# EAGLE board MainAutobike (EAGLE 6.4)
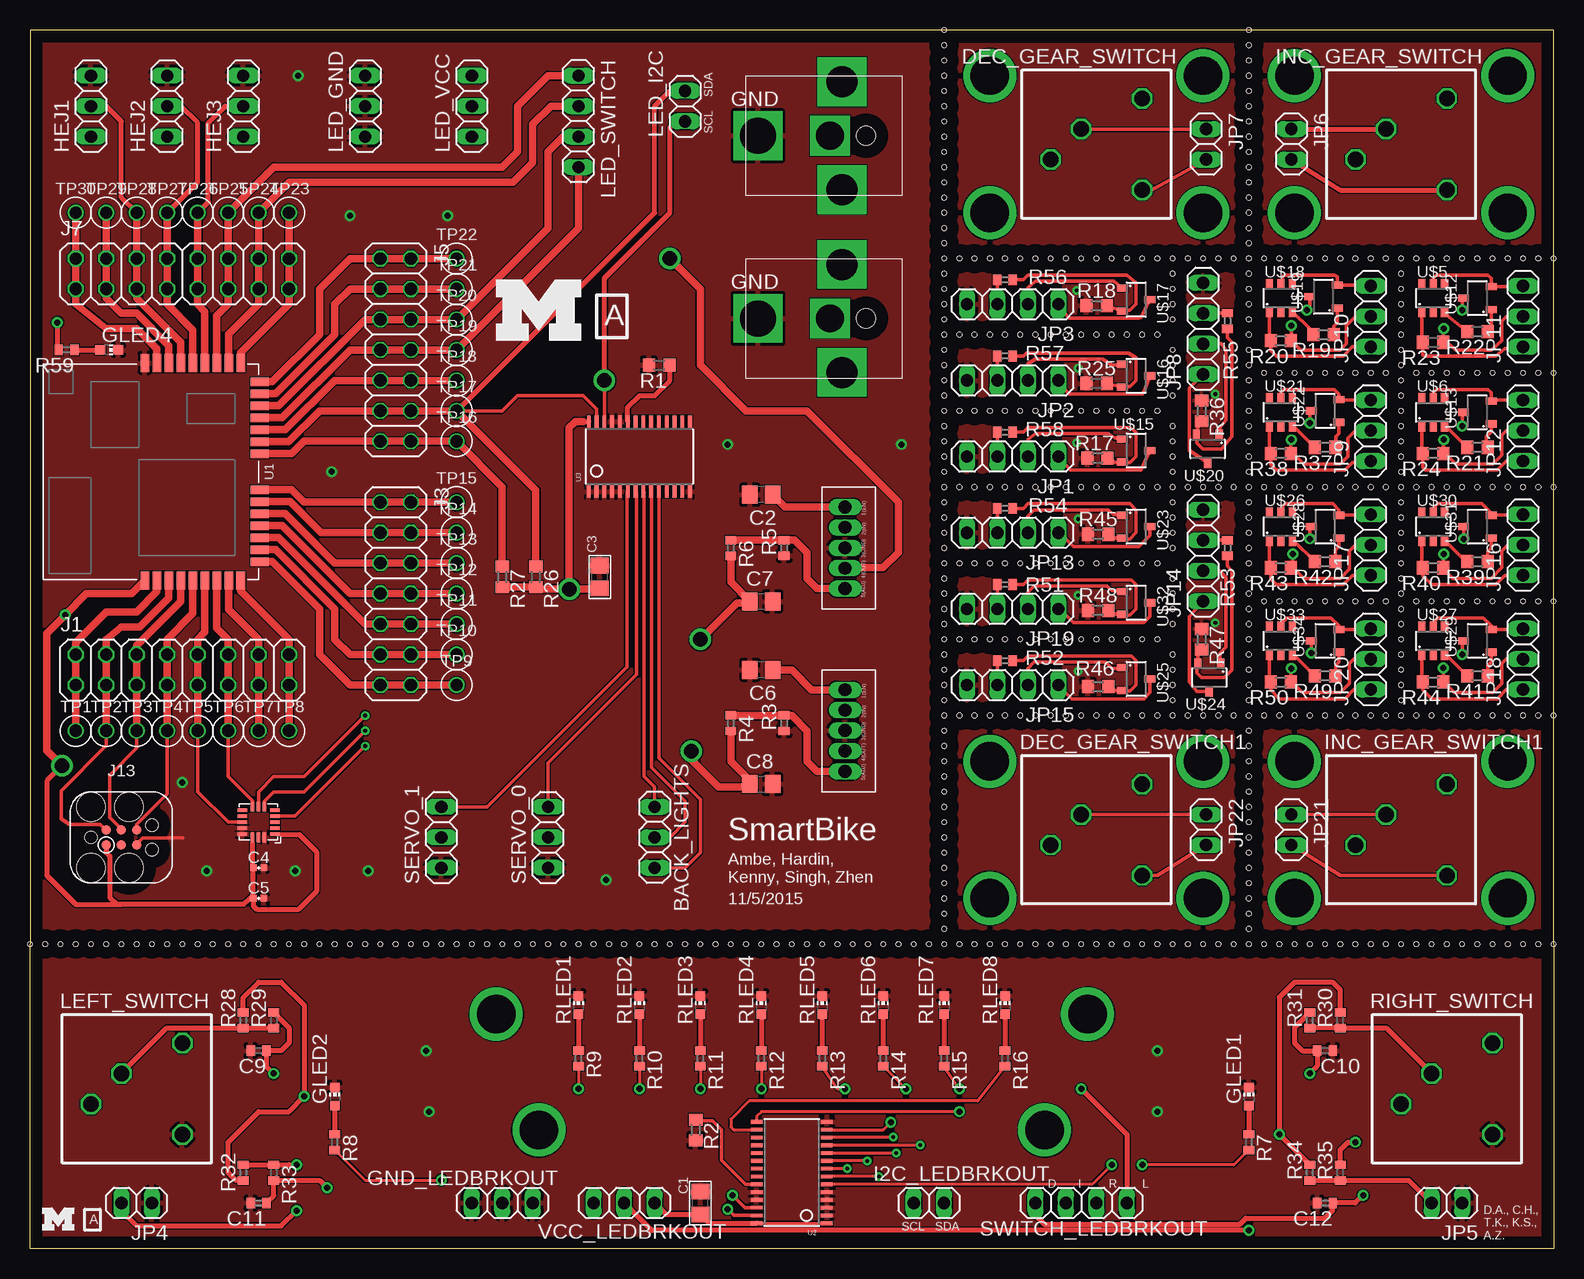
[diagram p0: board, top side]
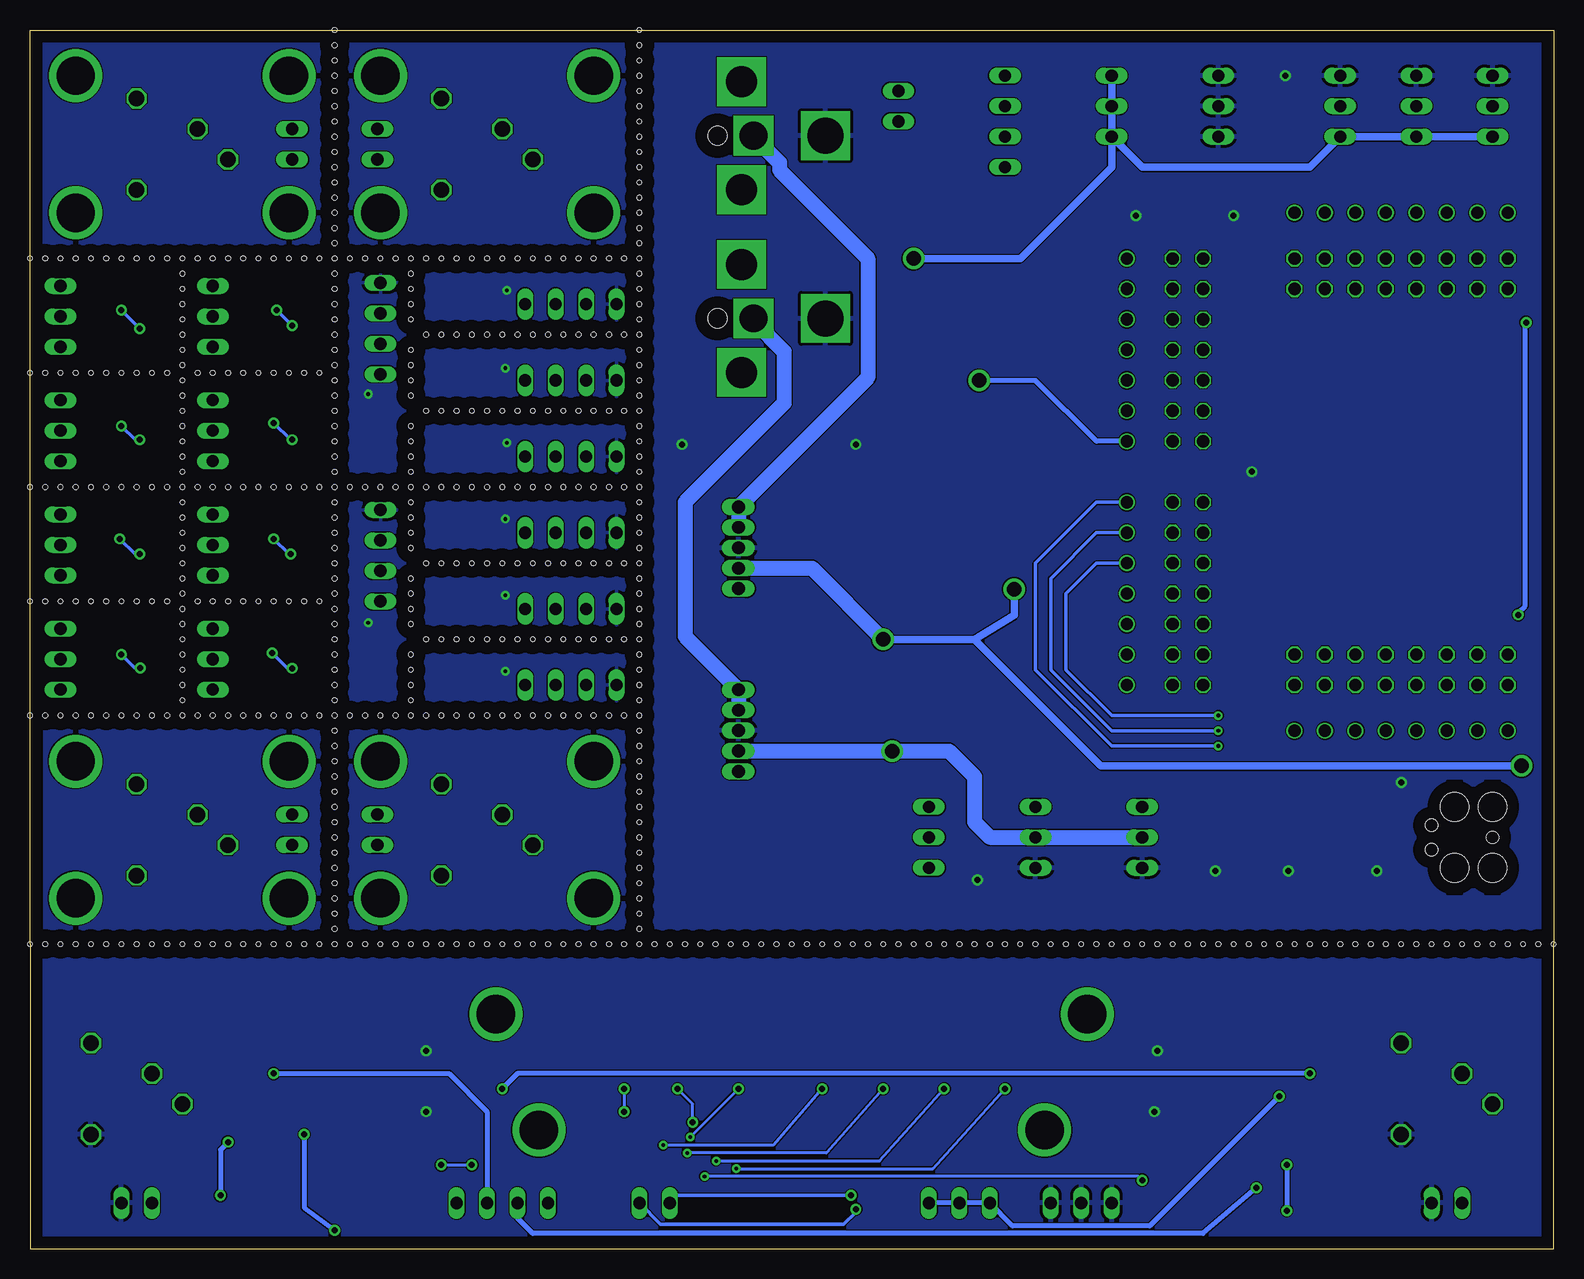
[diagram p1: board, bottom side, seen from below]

Size 127 x 101.6 mm. Coordinates in mm from the lower left corner, seen from the top.
Outline: 101.6,101.6 76.2,101.6 0,101.6 0,25.4 0,0 127,0 127,25.4 127,44.45 127,53.98 127,63.5 127,73.03 127,82.55 127,101.6 101.6,101.6
Copper layers (1*16): Top 0.035mm / dielectric 1.5mm / Bottom 0.035mm
Design rules "default *": minimum track width 4mil, minimum drill 12mil, track to track 4mil, track to pad 4mil, pad to pad 4mil, via to via 4mil, smd to smd 4mil, copper to edge 40mil, drill to drill 8mil, minimum pad ring 6mil, minimum via ring 8mil, stop-mask expansion 4mil, vias tented up to drill 0mil, thermal gap 10mil
Holes 0.38 mm at 0,25.4 1.27,25.4 2.54,25.4 3.81,25.4 5.08,25.4 6.35,25.4 7.62,25.4 8.89,25.4 10.16,25.4 11.43,25.4 12.7,25.4 13.97,25.4 15.24,25.4 16.51,25.4 17.78,25.4 19.05,25.4 20.32,25.4 21.59,25.4 22.86,25.4 24.13,25.4 25.4,25.4 26.67,25.4 27.94,25.4 29.21,25.4 30.48,25.4 31.75,25.4 33.02,25.4 34.29,25.4 35.56,25.4 36.83,25.4 38.1,25.4 39.37,25.4 40.64,25.4 41.91,25.4 43.18,25.4 44.45,25.4 45.72,25.4 46.99,25.4 48.26,25.4 49.53,25.4 50.8,25.4 52.07,25.4 53.34,25.4 54.61,25.4 55.88,25.4 57.15,25.4 58.42,25.4 59.69,25.4 60.96,25.4 62.23,25.4 63.5,25.4 64.77,25.4 66.04,25.4 67.31,25.4 68.58,25.4 69.85,25.4 71.12,25.4 72.39,25.4 73.66,25.4 74.93,25.4 76.2,25.4 77.47,25.4 78.74,25.4 80.01,25.4 81.28,25.4 82.55,25.4 83.82,25.4 85.09,25.4 86.36,25.4 87.63,25.4 88.9,25.4 90.17,25.4 91.44,25.4 92.71,25.4 93.98,25.4 95.25,25.4 96.52,25.4 97.79,25.4 99.06,25.4 100.33,25.4 101.6,25.4 102.87,25.4 104.14,25.4 105.41,25.4 106.68,25.4 107.95,25.4 109.22,25.4 110.49,25.4 111.76,25.4 113.03,25.4 114.3,25.4 115.57,25.4 116.84,25.4 118.11,25.4 119.38,25.4 120.65,25.4 121.92,25.4 123.19,25.4 124.46,25.4 125.73,25.4 127,25.4 76.2,101.6 76.2,100.33 76.2,99.06 76.2,97.79 76.2,96.52 76.2,95.25 76.2,93.98 76.2,92.71 76.2,91.44 76.2,90.17 76.2,88.9 76.2,87.63 76.2,86.36 76.2,85.09 76.2,83.82 76.2,82.55 76.2,81.28 76.2,80.01 76.2,78.74 76.2,77.47 76.2,76.2 76.2,74.93 76.2,73.66 76.2,72.39 76.2,71.12 76.2,69.85 76.2,68.58 76.2,67.31 76.2,66.04 76.2,64.77 76.2,63.5 76.2,62.23 76.2,60.96 76.2,59.69 76.2,58.42 76.2,57.15 76.2,55.88 76.2,54.61 76.2,53.34 76.2,52.07 76.2,50.8 76.2,49.53 76.2,48.26 76.2,46.99 76.2,45.72 76.2,44.45 76.2,43.18 76.2,41.91 76.2,40.64 76.2,39.37 76.2,38.1 76.2,36.83 76.2,35.56 76.2,34.29 76.2,33.02 76.2,31.75 76.2,30.48 76.2,29.21 76.2,27.94 76.2,26.67 101.6,101.6 101.6,100.33 101.6,99.06 101.6,97.79 101.6,96.52 101.6,95.25 101.6,93.98 101.6,92.71 101.6,91.44 101.6,90.17 101.6,88.9 101.6,87.63 101.6,86.36 101.6,85.09 101.6,83.82 101.6,81.28 101.6,80.01 101.6,78.74 101.6,77.47 101.6,76.2 101.6,74.93 101.6,73.66 101.6,72.39 101.6,71.12 101.6,69.85 101.6,68.58 101.6,67.31 101.6,66.04 101.6,64.77 101.6,63.5 101.6,62.23 101.6,60.96 101.6,59.69 101.6,58.42 101.6,57.15 101.6,55.88 101.6,54.61 101.6,53.34 101.6,52.07 101.6,50.8 101.6,49.53 101.6,48.26 101.6,46.99 101.6,45.72 101.6,44.45 101.6,43.18 101.6,41.91 101.6,40.64 101.6,39.37 101.6,38.1 101.6,36.83 101.6,35.56 101.6,34.29 101.6,33.02 101.6,31.75 101.6,30.48 101.6,29.21 101.6,27.94 101.6,26.67 77.47,44.45 78.74,44.45 80.01,44.45 81.28,44.45 82.55,44.45 83.82,44.45 85.09,44.45 86.36,44.45 87.63,44.45 88.9,44.45 90.17,44.45 91.44,44.45 92.71,44.45 93.98,44.45 95.25,44.45 96.52,44.45 97.79,44.45 99.06,44.45 100.33,44.45 102.87,44.45 104.14,44.45 105.41,44.45 106.68,44.45 107.95,44.45 109.22,44.45 110.49,44.45 111.76,44.45 113.03,44.45 114.3,44.45 115.57,44.45 116.84,44.45 118.11,44.45 119.38,44.45 120.65,44.45 121.92,44.45 123.19,44.45 124.46,44.45 125.73,44.45 77.47,63.5 78.74,63.5 80.01,63.5 81.28,63.5 82.55,63.5 83.82,63.5 85.09,63.5 86.36,63.5 87.63,63.5 88.9,63.5 90.17,63.5 91.44,63.5 92.71,63.5 93.98,63.5 95.25,63.5 96.52,63.5 97.79,63.5 99.06,63.5 100.33,63.5 102.87,63.5 104.14,63.5 105.41,63.5 106.68,63.5 107.95,63.5 109.22,63.5 110.49,63.5 111.76,63.5 113.03,63.5 114.3,63.5 115.57,63.5 116.84,63.5 118.11,63.5 119.38,63.5 120.65,63.5 121.92,63.5 123.19,63.5 124.46,63.5 125.73,63.5 101.6,82.55 77.47,82.55 78.74,82.55 80.01,82.55 81.28,82.55 82.55,82.55 83.82,82.55 85.09,82.55 86.36,82.55 87.63,82.55 88.9,82.55 90.17,82.55 91.44,82.55 92.71,82.55 93.98,82.55 95.25,82.55 96.52,82.55 97.79,82.55 99.06,82.55 100.33,82.55 102.87,82.55 104.14,82.55 105.41,82.55 106.68,82.55 107.95,82.55 109.22,82.55 110.49,82.55 111.76,82.55 113.03,82.55 114.3,82.55 115.57,82.55 116.84,82.55 118.11,82.55 119.38,82.55 120.65,82.55 121.92,82.55 123.19,82.55 124.46,82.55 125.73,82.55 77.47,69.85 78.74,69.85 80.01,69.85 81.28,69.85 82.55,69.85 83.82,69.85 85.09,69.85 86.36,69.85 87.63,69.85 88.9,69.85 90.17,69.85 91.44,69.85 92.71,69.85 93.98,69.85 95.25,67.31 95.25,66.04 95.25,64.77 95.25,71.12 95.25,72.39 95.25,73.66 95.25,74.93 95.25,68.58 93.98,76.2 95.25,77.47 95.25,78.74 95.25,80.01 95.25,81.28 77.47,76.2 78.74,76.2 80.01,76.2 81.28,76.2 82.55,76.2 83.82,76.2 85.09,76.2 86.36,76.2 87.63,76.2 88.9,76.2 90.17,76.2 91.44,76.2 92.71,76.2 102.87,73.03 104.14,73.03 105.41,73.03 106.68,73.03 107.95,73.03 109.22,73.03 110.49,73.03 111.76,73.03 113.03,73.03 114.3,81.28 114.3,80.01 114.3,78.74 114.3,77.47 114.3,76.2 114.3,74.93 114.3,73.66 115.57,73.03 116.84,73.03 118.11,73.03 119.38,73.03 120.65,73.03 121.92,73.03 123.19,73.03 124.46,73.03 125.73,73.03 114.3,72.39 114.3,71.12 114.3,69.85 114.3,68.58 114.3,67.31 114.3,66.04 114.3,64.77 114.3,62.23 114.3,60.96 114.3,59.69 114.3,58.42 114.3,57.15 114.3,55.88 114.3,54.61 114.3,53.34 114.3,52.07 114.3,50.8 114.3,49.53 114.3,48.26 114.3,46.99 114.3,45.72 102.87,53.98 104.14,53.98 105.41,53.98 106.68,53.98 107.95,53.98 109.22,53.98 110.49,53.98 111.76,53.98 113.03,53.98 115.57,53.98 116.84,53.98 118.11,53.98 119.38,53.98 120.65,53.98 121.92,53.98 123.19,53.98 124.46,53.98 125.73,53.98 95.25,48.26 95.25,46.99 95.25,45.72 95.25,52.07 95.25,53.34 95.25,54.61 95.25,55.88 95.25,49.53 95.25,58.42 95.25,59.69 95.25,60.96 95.25,62.23 77.47,57.15 78.74,57.15 80.01,57.15 81.28,57.15 82.55,57.15 83.82,57.15 85.09,57.15 86.36,57.15 87.63,57.15 88.9,57.15 90.17,57.15 91.44,57.15 92.71,57.15 93.98,57.15 77.47,50.8 78.74,50.8 80.01,50.8 81.28,50.8 82.55,50.8 83.82,50.8 85.09,50.8 86.36,50.8 87.63,50.8 88.9,50.8 90.17,50.8 91.44,50.8 92.71,50.8 93.98,50.8 127,82.55 127,73.03 127,63.5 127,53.98 127,44.45

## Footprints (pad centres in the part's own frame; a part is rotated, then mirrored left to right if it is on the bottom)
1X03 = drill 1.016 long: 1 -2.54,0; 2 0,0; 3 2.54,0
0805 = smd 1.3 x 1.5: 1 -0.95,0; 2 0.95,0
C0805 = smd 1.3 x 1.5: 1 -0.95,0; 2 0.95,0
0402_CAP = smd 0.536 x 0.546: 1 -0.433,0; 2 0.433,0
C0402 = smd 0.7 x 0.9: 1 -0.65,0; 2 0.65,0
LED_SWITCH = drill 1.3 octagon: P$1 -3.81,-1.27; P$2 -1.27,1.27; P$3 3.81,3.81; P$4 3.81,-3.81
CHIP-LED0603 = smd 0.8 x 0.8: A 0,-0.75; C 0,0.75
1X02 = drill 1.016 long: 1 -1.27,0; 2 1.27,0
2X08 = drill 1.016 octagon: 1 -8.89,-1.27; 2 -8.89,1.27; 3 -6.35,-1.27; 4 -6.35,1.27; 5 -3.81,-1.27; 6 -3.81,1.27; 7 -1.27,-1.27; 8 -1.27,1.27; 9 1.27,-1.27; 10 1.27,1.27; 11 3.81,-1.27; 12 3.81,1.27; 13 6.35,-1.27; 14 6.35,1.27; 15 8.89,-1.27; 16 8.89,1.27
2X07 = drill 1.016 octagon: 1 -7.62,-1.27; 2 -7.62,1.27; 3 -5.08,-1.27; 4 -5.08,1.27; 5 -2.54,-1.27; 6 -2.54,1.27; 7 0,-1.27; 8 0,1.27; 9 2.54,-1.27; 10 2.54,1.27; 11 5.08,-1.27; 12 5.08,1.27; 13 7.62,-1.27; 14 7.62,1.27
TC2030-IDC = smd 0.787 x 0.787: 1 -1.27,-0.635; 2 -1.27,0.635; 3 0,-0.635; 4 0,0.635; 5 1.27,-0.635; 6 1.27,0.635 | hole 2.375: -2.54,2.54; 0.635,2.54; 0.635,-2.54; -2.54,-2.54 | hole 1.016: -2.54,0; 2.54,1.016; 2.54,-1.016
1X04 = drill 1.016 long: 1 -3.81,0; 2 -1.27,0; 3 1.27,0; 4 3.81,0
R0603 = smd 1 x 1.1: 1 -0.85,0; 2 0.85,0
R0402 = smd 0.7 x 0.9: 1 -0.65,0; 2 0.65,0
TESTPOINT_0.040IN = drill 1.016: TESTPOINT 0,0
ATUM = smd 0.7 x 1.5: 1 -9.479,-9.079; 2 -8.479,-9.079; 3 -7.479,-9.079; 4 -6.479,-9.079; 5 -5.479,-9.079; 6 -4.479,-9.079; 7 -3.479,-9.079; 8 -2.479,-9.079; 24 -1.479,9.079; 25 -2.479,9.079; 26 -3.479,9.079; 27 -4.479,9.079; 28 -5.479,9.079; 29 -6.479,9.079; 30 -7.479,9.079; 31 -8.479,9.079; 32 -9.479,9.079 | smd 0.754 x 1.5: 9 -1.479,-9.079 | smd 1.5 x 0.7: 10 0.1,-7.5; 11 0.1,-6.5; 12 0.1,-5.5; 13 0.1,-4.5; 14 0.1,-3.5; 15 0.1,-2.5; 16 0.1,-1.5; 17 0.1,1.5; 18 0.1,2.5; 19 0.1,3.5; 20 0.1,4.5; 21 0.1,5.5; 22 0.1,6.5; 23 0.1,7.5
TSSOP28 = smd 0.305 x 0.991: 1 -4.225,-2.918; 2 -3.575,-2.918; 3 -2.925,-2.918; 4 -2.275,-2.918; 5 -1.625,-2.918; 6 -0.975,-2.918; 7 -0.325,-2.918; 8 0.325,-2.918; 9 0.975,-2.918; 10 1.625,-2.918; 11 2.275,-2.918; 12 2.925,-2.918; 13 3.575,-2.918; 14 4.225,-2.918; 15 4.225,2.918; 16 3.575,2.918; 17 2.925,2.918; 18 2.275,2.918; 19 1.625,2.918; 20 0.975,2.918; 21 0.325,2.918; 22 -0.325,2.918; 23 -0.975,2.918; 24 -1.625,2.918; 25 -2.275,2.918; 26 -2.925,2.918; 27 -3.575,2.918; 28 -4.225,2.918
ADXL362 = smd 0.8 x 0.3: P$1 -1.35,1; P$2 -1.35,0.5; P$3 -1.35,0; P$4 -1.35,-0.5; P$5 -1.35,-1; P$9 1.35,-1; P$10 1.35,-0.5; P$11 1.35,0; P$12 1.35,0.5; P$13 1.35,1 | smd 0.3 x 0.8: P$6 -0.5,-1.275; P$7 0,-1.275; P$8 0.5,-1.275; P$14 0.5,1.275; P$15 0,1.275; P$16 -0.5,1.275
MIC29710 = drill 1.067 pad 1.27 long: 1(EN) 1.664,1.905; 2(IN) 3.365,1.905; 3(GND) 5.067,1.905; 4(OUT) 6.769,1.905; 5(ADJ) 8.471,1.905
SOT23-6 = smd 0.6 x 0.9: 1 -0.95,-1.15; 2 0,-1.15; 3 0.95,-1.15; 4 0.95,1.15; 5 0,1.15; 6 -0.95,1.15
PJ063BH = drill 2.6 pad 4.064 square: FRAME0 0.5,8; FRAME1 9.5,8 | drill 3 pad 4.064 square: GND 5,1 | drill 2.3 pad 3.302 square: VDD 5,7 | hole 1.6: 5,10
SOT23-3 = smd 0.6 x 0.9: 1 -0.95,-1.15; 2 0.95,-1.15; 3 0,1.15

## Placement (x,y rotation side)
BACK_LIGHTS  [1X03]  52.07,34.29 270 top
C1  10uF  [0805]  55.88,3.81 90 top
C2  10uF  [C0805]  60.96,62.87 180 top
C3  10uF  [0805]  47.5,56.01 90 top
C4  100nF  [0402_CAP]  19.05,31.75 0 top
C5  100nF  [0402_CAP]  19.05,29.21 0 top
C6  10uF  [C0805]  60.96,48.26 180 top
C7  33uF  [C0805]  60.96,53.98 0 top
C8  33uF  [C0805]  60.96,38.73 0 top
C9  [C0402]  19.05,16.51 180 top
C10  [C0402]  107.95,16.51 0 top
C11  [C0402]  19.05,3.81 180 top
C12  [C0402]  107.95,3.81 180 top
DEC_GEAR_SWITCH  LED_SWITCH  [LED_SWITCH]  88.9,92.08 0 top
DEC_GEAR_SWITCH1  LED_SWITCH  [LED_SWITCH]  88.9,34.92 0 top
GLED1  [CHIP-LED0603]  101.6,12.7 0 top
GLED2  [CHIP-LED0603]  25.4,12.7 0 top
GLED4  [CHIP-LED0603]  6.6,74.93 270 top
GND_LEDBRKOUT  [1X03]  39.37,3.81 0 top
HEJ1  [1X03]  5.08,95.25 90 top
HEJ2  [1X03]  11.43,95.25 90 top
HEJ3  [1X03]  17.78,95.25 90 top
I2C_LEDBRKOUT  [1X02]  74.93,3.81 0 top
INC_GEAR_SWITCH  LED_SWITCH  [LED_SWITCH]  114.3,92.08 0 top
INC_GEAR_SWITCH1  LED_SWITCH  [LED_SWITCH]  114.3,34.92 0 top
J1  [2X08]  12.7,48.26 0 top
J3  [2X07]  30.48,54.61 270 top
J5  [2X07]  30.48,74.93 270 top
J7  [2X08]  12.7,81.28 0 top
J13  TC2030-CTX  [TC2030-IDC]  7.62,34.29 0 top
JP1  [1X04]  81.91,66.04 180 top
JP2  [1X04]  81.91,72.39 180 top
JP3  [1X04]  81.91,78.74 180 top
JP4  [1X02]  8.89,3.81 180 top
JP5  [1X02]  118.11,3.81 180 top
JP6  [1X02]  105.16,92.08 270 top
JP7  [1X02]  98.04,92.08 270 top
JP8  [1X04]  97.79,76.71 90 top
JP9  [1X03]  111.76,68.2 90 top
JP10  [1X03]  111.76,77.72 90 top
JP11  [1X03]  124.46,77.72 90 top
JP12  [1X03]  124.46,68.2 90 top
JP13  [1X04]  81.91,59.69 180 top
JP14  [1X04]  97.79,57.78 90 top
JP15  [1X04]  81.91,46.99 180 top
JP16  [1X03]  124.46,58.67 90 top
JP17  [1X03]  111.76,58.67 90 top
JP18  [1X03]  124.46,49.15 90 top
JP19  [1X04]  81.91,53.34 180 top
JP20  [1X03]  111.76,49.15 90 top
JP21  [1X02]  105.16,34.92 270 top
JP22  [1X02]  98.04,34.92 270 top
LED_GND  [1X03]  27.94,95.25 90 top
LED_I2C  [1X02]  54.61,95.25 90 top
LED_SWITCH  [1X04]  45.72,93.98 270 top
LED_VCC  [1X03]  36.83,95.25 90 top
LEFT_SWITCH  LED_SWITCH  [LED_SWITCH]  8.89,13.34 0 top
R1  10K  [R0603]  52.45,73.66 180 top
R2  10K  [R0603]  55.5,9.91 270 top
R3  26.1k  [R0402]  62.87,43.81 90 top
R4  100k  [R0402]  58.42,43.81 270 top
R5  60.4k  [R0402]  62.87,58.42 90 top
R6  100k  [R0402]  58.42,58.42 270 top
R7  60.4  [R0402]  101.6,8.89 270 top
R8  60.4  [R0402]  25.4,8.89 270 top
R9  261  [R0402]  45.72,15.88 270 top
R10  261  [R0402]  50.8,15.88 270 top
R11  261  [R0402]  55.88,15.88 270 top
R12  261  [R0402]  60.96,15.88 270 top
R13  261  [R0402]  66.04,15.88 270 top
R14  261  [R0402]  71.12,15.88 270 top
R15  261  [R0402]  76.2,15.88 270 top
R16  261  [R0402]  81.28,15.88 270 top
R17  10k  [R0603]  88.98,65.91 0 top
R18  10k  [R0603]  88.9,78.61 0 top
R19  1k  [R0603]  107.82,76.2 180 top
R20  390  [R0603]  104.27,75.69 180 top
R21  1k  [R0603]  120.65,66.8 180 top
R22  1k  [R0603]  120.65,76.45 180 top
R23  390  [R0603]  116.97,75.56 180 top
R24  390  [R0603]  116.97,66.29 180 top
R25  10k  [R0603]  88.9,72.14 0 top
R26  10k  [R0603]  42.16,56.01 270 top
R27  10k  [R0603]  39.37,56.01 270 top
R28  [R0402]  17.78,19.05 90 top
R29  [R0402]  20.32,19.05 90 top
R30  [R0402]  109.22,19.05 90 top
R31  [R0402]  106.68,19.05 90 top
R32  [R0402]  17.78,6.35 270 top
R33  [R0402]  20.32,6.35 270 top
R34  [R0402]  106.68,6.35 90 top
R35  [R0402]  109.22,6.35 90 top
R36  10k  [R0603]  97.66,69.85 270 top
R37  1k  [R0603]  107.95,66.8 180 top
R38  390  [R0603]  104.27,66.29 180 top
R39  1k  [R0603]  120.65,57.28 180 top
R40  390  [R0603]  116.97,56.77 180 top
R41  1k  [R0603]  120.65,47.75 180 top
R42  1k  [R0603]  107.95,57.28 180 top
R43  390  [R0603]  104.27,56.77 180 top
R44  390  [R0603]  116.97,47.24 180 top
R45  10k  [R0603]  89.03,59.56 0 top
R46  10k  [R0603]  89.03,46.86 0 top
R47  10k  [R0603]  97.66,50.8 270 top
R48  10k  [R0603]  89.03,53.21 0 top
R49  1k  [R0603]  107.95,47.75 180 top
R50  390  [R0603]  104.27,47.24 180 top
R51  33  [R0402]  81.28,55.37 0 top
R52  33  [R0402]  81.28,49.02 0 top
R53  33  [R0402]  99.82,58.42 270 top
R54  33  [R0402]  81.28,61.72 0 top
R55  33  [R0402]  99.82,77.34 270 top
R56  33  [R0402]  81.28,80.77 0 top
R57  33  [R0402]  81.28,74.42 0 top
R58  33  [R0402]  81.28,68.07 0 top
R59  60.4  [R0402]  3.05,74.93 180 top
RIGHT_SWITCH  LED_SWITCH  [LED_SWITCH]  118.11,13.34 0 top
RLED1  [CHIP-LED0603]  45.72,20.32 0 top
RLED2  [CHIP-LED0603]  50.8,20.32 0 top
RLED3  [CHIP-LED0603]  55.88,20.32 0 top
RLED4  [CHIP-LED0603]  60.96,20.32 0 top
RLED5  [CHIP-LED0603]  66.04,20.32 0 top
RLED6  [CHIP-LED0603]  71.12,20.32 0 top
RLED7  [CHIP-LED0603]  76.2,20.32 0 top
RLED8  [CHIP-LED0603]  81.28,20.32 0 top
SERVO_0  [1X03]  43.18,34.29 90 top
SERVO_1  [1X03]  34.29,34.29 90 top
SWITCH_LEDBRKOUT  [1X04]  87.63,3.81 0 top
TP1  TEST_POINT_0.040IN  [TESTPOINT_0.040IN]  3.81,43.18 0 top
TP2  TEST_POINT_0.040IN  [TESTPOINT_0.040IN]  6.35,43.18 0 top
TP3  TEST_POINT_0.040IN  [TESTPOINT_0.040IN]  8.89,43.18 0 top
TP4  TEST_POINT_0.040IN  [TESTPOINT_0.040IN]  11.43,43.18 0 top
TP5  TEST_POINT_0.040IN  [TESTPOINT_0.040IN]  13.97,43.18 0 top
TP6  TEST_POINT_0.040IN  [TESTPOINT_0.040IN]  16.51,43.18 0 top
TP7  TEST_POINT_0.040IN  [TESTPOINT_0.040IN]  19.05,43.18 0 top
TP8  TEST_POINT_0.040IN  [TESTPOINT_0.040IN]  21.59,43.18 0 top
TP9  TEST_POINT_0.040IN  [TESTPOINT_0.040IN]  35.56,46.99 0 top
TP10  TEST_POINT_0.040IN  [TESTPOINT_0.040IN]  35.56,49.53 0 top
TP11  TEST_POINT_0.040IN  [TESTPOINT_0.040IN]  35.56,52.07 0 top
TP12  TEST_POINT_0.040IN  [TESTPOINT_0.040IN]  35.56,54.61 0 top
TP13  TEST_POINT_0.040IN  [TESTPOINT_0.040IN]  35.56,57.15 0 top
TP14  TEST_POINT_0.040IN  [TESTPOINT_0.040IN]  35.56,59.69 0 top
TP15  TEST_POINT_0.040IN  [TESTPOINT_0.040IN]  35.56,62.23 0 top
TP16  TEST_POINT_0.040IN  [TESTPOINT_0.040IN]  35.56,67.31 0 top
TP17  TEST_POINT_0.040IN  [TESTPOINT_0.040IN]  35.56,69.85 0 top
TP18  TEST_POINT_0.040IN  [TESTPOINT_0.040IN]  35.56,72.39 0 top
TP19  TEST_POINT_0.040IN  [TESTPOINT_0.040IN]  35.56,74.93 0 top
TP20  TEST_POINT_0.040IN  [TESTPOINT_0.040IN]  35.56,77.47 0 top
TP21  TEST_POINT_0.040IN  [TESTPOINT_0.040IN]  35.56,80.01 0 top
TP22  TEST_POINT_0.040IN  [TESTPOINT_0.040IN]  35.56,82.55 0 top
TP23  TEST_POINT_0.040IN  [TESTPOINT_0.040IN]  21.59,86.36 0 top
TP24  TEST_POINT_0.040IN  [TESTPOINT_0.040IN]  19.05,86.36 0 top
TP25  TEST_POINT_0.040IN  [TESTPOINT_0.040IN]  16.51,86.36 0 top
TP26  TEST_POINT_0.040IN  [TESTPOINT_0.040IN]  13.97,86.36 0 top
TP27  TEST_POINT_0.040IN  [TESTPOINT_0.040IN]  11.43,86.36 0 top
TP28  TEST_POINT_0.040IN  [TESTPOINT_0.040IN]  8.89,86.36 0 top
TP29  TEST_POINT_0.040IN  [TESTPOINT_0.040IN]  6.35,86.36 0 top
TP30  TEST_POINT_0.040IN  [TESTPOINT_0.040IN]  3.81,86.36 0 top
U1  ATUM  [ATUM]  19.05,64.77 0 top
U2  PCA9685  [TSSOP28]  63.5,6.35 90 top
U3  PCA9685  [TSSOP28]  50.8,66.04 0 top
U4  ADXL362  [ADXL362]  19.05,35.56 180 top
U$1  [UMICH_SOLID_200MIL]  38.86,75.69 0 top
U$2  MIC29710  [MIC29710]  66.04,63.5 270 top
U$3  [UMICH_SOLID_75MIL]  1.02,1.52 0 top
U$4  MIC29710  [MIC29710]  66.04,48.26 270 top
U$5  HALLEFFECT  [SOT23-6]  116.97,79.25 0 top
U$6  HALLEFFECT  [SOT23-6]  116.97,69.72 0 top
U$11  PJ063PH  [PJ063BH]  59.69,97.79 270 top
U$12  25AA02E48-SOT-23-6  [SOT23-3]  120.65,79.25 90 top
U$13  25AA02E48-SOT-23-6  [SOT23-3]  120.65,69.72 90 top
U$14  PJ063PH  [PJ063BH]  59.69,82.55 270 top
U$15  25AA02E48-SOT-23-6  [SOT23-3]  92.2,66.55 270 top
U$16  25AA02E48-SOT-23-6  [SOT23-3]  92.2,72.77 270 top
U$17  25AA02E48-SOT-23-6  [SOT23-3]  92.2,79.12 270 top
U$18  HALLEFFECT  [SOT23-6]  104.27,79.25 0 top
U$19  25AA02E48-SOT-23-6  [SOT23-3]  107.82,79.38 90 top
U$20  25AA02E48-SOT-23-6  [SOT23-3]  98.17,66.67 180 top
U$21  HALLEFFECT  [SOT23-6]  104.27,69.72 0 top
U$22  25AA02E48-SOT-23-6  [SOT23-3]  107.95,69.85 90 top
U$23  25AA02E48-SOT-23-6  [SOT23-3]  92.2,60.2 270 top
U$24  25AA02E48-SOT-23-6  [SOT23-3]  98.3,47.62 180 top
U$25  25AA02E48-SOT-23-6  [SOT23-3]  92.2,47.5 270 top
U$26  HALLEFFECT  [SOT23-6]  104.27,60.2 0 top
U$27  HALLEFFECT  [SOT23-6]  116.97,50.67 0 top
U$28  25AA02E48-SOT-23-6  [SOT23-3]  107.95,60.2 90 top
U$29  25AA02E48-SOT-23-6  [SOT23-3]  120.65,50.67 90 top
U$30  HALLEFFECT  [SOT23-6]  116.97,60.2 0 top
U$31  25AA02E48-SOT-23-6  [SOT23-3]  120.65,60.2 90 top
U$32  25AA02E48-SOT-23-6  [SOT23-3]  92.2,53.85 270 top
U$33  HALLEFFECT  [SOT23-6]  104.27,50.67 0 top
U$34  25AA02E48-SOT-23-6  [SOT23-3]  107.95,50.67 90 top
VCC_LEDBRKOUT  [1X03]  49.53,3.81 0 top

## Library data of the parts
BACK_LIGHTS GND_LEDBRKOUT HEJ1-HEJ3 I2C_LEDBRKOUT JP1-JP22 LED_GND LED_I2C LED_SWITCH LED_VCC SERVO_0 SERVO_1 SWITCH_LEDBRKOUT VCC_LEDBRKOUT = pinhead
C1 C3 U2 U3 = microbuilder
C2 C6-C12 R1-R59 = rcl
C4 C5 = passives
DEC_GEAR_SWITCH DEC_GEAR_SWITCH1 INC_GEAR_SWITCH INC_GEAR_SWITCH1 LEFT_SWITCH RIGHT_SWITCH = led_switch
GLED1 GLED2 GLED4 RLED1-RLED8 = led
J1 J7 = pinhead; DIGIKEY: 609-3364-ND; MOUSER: 649-68602-116HLF; NEWARK: 20M2833
J3 J5 = pinhead; DIGIKEY: 609-3491-ND; MOUSER: 649-67996-114HLF; NEWARK: 30M1973
J13 = connector
TP1-TP30 = headers; DIGIKEY: 5001K-ND
U1 = atum
U4 = SparkFun-Sensors
U$1 U$3 = logos
U$2 U$4 = MIC29710_new2
U$5 U$6 U$12 U$13 U$15-U$34 = 25AA02E48
U$11 U$14 = PJ063PH

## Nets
19: LEFT_SWITCH.P$2 R28.1 R29.1
20: R30.1 R31.1 RIGHT_SWITCH.P$2
21: JP4.2 R32.1 R33.1
22: JP5.2 R34.1 R35.1
!RESET: J7.3 J7.4 TP29.TESTPOINT U1.30
AIN3: J7.13 J7.14 LED_SWITCH.2 TP24.TESTPOINT U1.25
AIN4: J7.11 J7.12 LED_SWITCH.1 TP25.TESTPOINT U1.26
AIN5: HEJ3.2 J7.9 J7.10 TP26.TESTPOINT U1.27
AIN6: HEJ2.2 J7.7 J7.8 TP27.TESTPOINT U1.28
AIN7: HEJ1.2 J7.5 J7.6 TP28.TESTPOINT U1.29
BATTERY: J7.1 J7.2 TP30.TESTPOINT U1.31
BOOTLOADER_CTRL: J7.15 J7.16 TP23.TESTPOINT U1.24
BOOTLOADER_RX: J5.3 J5.4 TP21.TESTPOINT U1.22
BOOTLOADER_TX: J5.1 J5.2 TP22.TESTPOINT U1.23
DEC_GEAR_SWITCH_OUT: C12.1 R35.2 SWITCH_LEDBRKOUT.1
DGND_USB: J3.13 J3.14 TP9.TESTPOINT U1.10
DVDD_USB: J3.7 J3.8 TP12.TESTPOINT U1.13
GND: C2.2 C3.2 C4.2 C5.2 C6.2 C7.2 C8.2 GLED4.C HEJ1.3 HEJ2.3 HEJ3.3 J13.5 LED_GND.1 LED_GND.2 LED_GND.3 R1.2 R3.1 R5.1 SERVO_0.1 SERVO_1.1 U1.32 U3.1 U3.2 U3.3 U3.4 U3.5 U3.14 U3.24 U3.25 U4.P$12 U4.P$13 U4.P$16 U$2.3(GND) U$4.3(GND) U$11.GND U$14.GND
GND_LEDBRKOUT: C1.2 C9.2 C10.2 C11.2 C12.2 GLED1.C GLED2.C GND_LEDBRKOUT.1 GND_LEDBRKOUT.2 GND_LEDBRKOUT.3 JP4.1 JP5.1 LEFT_SWITCH.P$4 R2.2 RIGHT_SWITCH.P$4 RLED1.C RLED2.C RLED3.C RLED4.C RLED5.C RLED6.C RLED7.C RLED8.C U2.2 U2.3 U2.4 U2.5 U2.14 U2.24 U2.25
GND_LGT1: JP1.4 R17.1
GND_LGT2: JP2.4 R25.1
GND_LGT3: JP3.4 R18.1
GND_LGT4: JP8.4 R36.1
GND_LGT5: JP13.4 R45.1
GND_LGT6: JP14.4 R47.1
GND_LGT7: JP15.4 R46.1
GND_LGT8: JP19.4 R48.1
HE1GND: JP10.3 U$18.5 U$19.2
HE1OUT: JP10.2 R20.1 U$19.3
HE1VIN: JP10.1 R20.2 U$18.1
HE2GND: JP11.3 U$5.5 U$12.2
HE2OUT: JP11.2 R23.1 U$12.3
HE2VIN: JP11.1 R23.2 U$5.1
HE3GND: JP12.3 U$6.5 U$13.2
HE3OUT: JP12.2 R24.1 U$13.3
HE3VIN: JP12.1 R24.2 U$6.1
HE4GND: JP9.3 U$21.5 U$22.2
HE4OUT: JP9.2 R38.1 U$22.3
HE4VIN: JP9.1 R38.2 U$21.1
HE5GND: JP16.3 U$30.5 U$31.2
HE5OUT: JP16.2 R40.1 U$31.3
HE5VIN: JP16.1 R40.2 U$30.1
HE6GND: JP17.3 U$26.5 U$28.2
HE6OUT: JP17.2 R43.1 U$28.3
HE6VIN: JP17.1 R43.2 U$26.1
HE7GND: JP18.3 U$27.5 U$29.2
HE7OUT: JP18.2 R44.1 U$29.3
HE7VIN: JP18.1 R44.2 U$27.1
HE8GND: JP20.3 U$33.5 U$34.2
HE8OUT: JP20.2 R50.1 U$34.3
HE8VIN: JP20.1 R50.2 U$33.1
I2C_SCL: J5.13 J5.14 LED_I2C.1 R27.1 TP16.TESTPOINT U1.17 U3.26
I2C_SCL_LEDBRKOUT: I2C_LEDBRKOUT.1 U2.26
I2C_SDA: J5.11 J5.12 LED_I2C.2 R26.1 TP17.TESTPOINT U1.18 U3.27
I2C_SDA_LEDBRKOUT: I2C_LEDBRKOUT.2 U2.27
INC_GEAR_SWITCH_OUT: C11.1 R33.2 SWITCH_LEDBRKOUT.2
LEFT_SWITCH_OUT: C9.1 R29.2 SWITCH_LEDBRKOUT.4
N$1: R16.1 RLED8.A
N$2: R5.2 R6.1 U$2.5(ADJ)
N$3: R3.2 R4.1 U$4.5(ADJ)
N$4: R15.1 RLED7.A
N$5: R14.1 RLED6.A
N$6: R13.1 RLED5.A
N$7: R12.1 RLED4.A
N$8: R11.1 RLED3.A
N$9: R10.1 RLED2.A
N$10: R9.1 RLED1.A
N$11: GLED2.A R8.1
N$12: GLED1.A R7.1
N$13: R37.1 U$22.1
N$14: R37.2 U$21.3
N$15: R19.1 U$19.1
N$16: R19.2 U$18.3
N$17: R39.1 U$31.1
N$18: R21.1 U$13.1
N$19: R39.2 U$30.3
N$20: R41.1 U$29.1
N$21: R21.2 U$6.3
N$22: R41.2 U$27.3
N$23: R42.1 U$28.1
N$24: R22.1 U$12.1
N$25: R22.2 U$5.3
N$26: R42.2 U$26.3
N$27: R49.1 U$34.1
N$28: R49.2 U$33.3
N$29: JP19.3 R51.1
N$30: JP15.3 R52.1
N$31: JP14.3 R53.1
N$32: JP13.3 R54.1
N$33: JP8.3 R55.1
N$34: JP3.3 R56.1
N$35: INC_GEAR_SWITCH.P$4 JP6.2
N$36: INC_GEAR_SWITCH.P$2 JP6.1
N$37: DEC_GEAR_SWITCH.P$4 JP7.2
N$38: DEC_GEAR_SWITCH.P$2 JP7.1
N$39: JP2.3 R57.1
N$42: JP1.3 R58.1
N$43: INC_GEAR_SWITCH1.P$4 JP21.2
N$44: INC_GEAR_SWITCH1.P$2 JP21.1
N$45: DEC_GEAR_SWITCH1.P$4 JP22.2
N$49: DEC_GEAR_SWITCH1.P$2 JP22.1
N$79: GLED4.A R59.1
OE: R1.1 U3.23
OE_LEDBRKOUT: R2.1 U2.23
OUT_LGT1: R17.2 R58.2 U$15.2
OUT_LGT2: R25.2 R57.2 U$16.2
OUT_LGT3: R18.2 R56.2 U$17.2
OUT_LGT4: R36.2 R55.2 U$20.2
OUT_LGT5: R45.2 R54.2 U$23.2
OUT_LGT6: R47.2 R53.2 U$24.2
OUT_LGT7: R46.2 R52.2 U$25.2
OUT_LGT8: R48.2 R51.2 U$32.2
P08: J5.9 J5.10 TP18.TESTPOINT U1.19
P09: J5.7 J5.8 LED_SWITCH.4 TP19.TESTPOINT U1.20
P10: J5.5 J5.6 LED_SWITCH.3 TP20.TESTPOINT U1.21
P17: J1.1 J1.2 TP1.TESTPOINT U1.2
P21: J1.9 J1.10 TP5.TESTPOINT U1.6 U4.P$11
P22: J1.11 J1.12 TP6.TESTPOINT U1.7 U4.P$8
P23: J1.13 J1.14 TP7.TESTPOINT U1.8
P24: J1.15 J1.16 TP8.TESTPOINT U1.9
PWM0: SERVO_1.3 U3.6
PWM0_0: R7.2 U2.6
PWM1: SERVO_0.3 U3.7
PWM1_0: R8.2 U2.7
PWM2: BACK_LIGHTS.1 U3.8
PWM2_0: R9.2 U2.8
PWM3: BACK_LIGHTS.2 U3.9
PWM3_0: R10.2 U2.9
PWM4: BACK_LIGHTS.3 U3.10
PWM4_0: R11.2 U2.10
PWM5: U3.11
PWM5_0: R12.2 U2.11
PWM6: U3.12
PWM6_0: R13.2 U2.12
PWM7: U3.13
PWM7_0: R14.2 U2.13
PWM8: U3.15
PWM8_0: R15.2 U2.15
PWM9: U3.16
PWM9_0: R16.2 U2.16
PWM10: U3.17
PWM10_0: U2.17
PWM11: U3.18
PWM11_0: U2.18
PWM12: U3.19
PWM12_0: U2.19
PWM13: U3.20
PWM13_0: U2.20
PWM14: U3.21
PWM14_0: U2.21
PWM15: U3.22
PWM15_0: U2.22
RIGHT_SWITCH_OUT: C10.1 R31.2 SWITCH_LEDBRKOUT.3
SIG_LGT1: JP1.2 U$15.1
SIG_LGT2: JP2.2 U$16.1
SIG_LGT3: JP3.2 U$17.1
SIG_LGT4: JP8.2 U$20.1
SIG_LGT5: JP13.2 U$23.1
SIG_LGT6: JP14.2 U$24.1
SIG_LGT7: JP15.2 U$25.1
SIG_LGT8: JP19.2 U$32.1
SPI_MISO: J3.5 J3.6 TP13.TESTPOINT U1.14 U4.P$7
SPI_MOSI: J3.3 J3.4 TP14.TESTPOINT U1.15 U4.P$6
SPI_SCK: J3.1 J3.2 TP15.TESTPOINT U1.16 U4.P$4
TCK: J1.5 J1.6 J13.4 TP3.TESTPOINT U1.4
TDO: J1.7 J1.8 J13.6 TP4.TESTPOINT U1.5
TMS: J1.3 J1.4 J13.2 TP2.TESTPOINT U1.3
USB_N: J3.9 J3.10 TP11.TESTPOINT U1.12
USB_P: J3.11 J3.12 TP10.TESTPOINT U1.11
VCC(3.3V): C3.1 C4.1 C5.1 C7.1 HEJ1.1 HEJ2.1 HEJ3.1 J13.1 LED_VCC.1 LED_VCC.2 LED_VCC.3 R6.2 R26.2 R27.2 R59.2 U1.1 U3.28 U4.P$1 U4.P$14 U$2.4(OUT)
VCC(6V): C8.1 R4.2 SERVO_0.2 SERVO_1.2 U$4.4(OUT)
VCC_LEDBRKOUT: C1.1 R28.2 R30.2 R32.2 R34.2 U2.1 U2.28 VCC_LEDBRKOUT.1 VCC_LEDBRKOUT.2 VCC_LEDBRKOUT.3
VCC_LGT1: JP1.1 U$15.3
VCC_LGT2: JP2.1 U$16.3
VCC_LGT3: JP3.1 U$17.3
VCC_LGT4: JP8.1 U$20.3
VCC_LGT5: JP13.1 U$23.3
VCC_LGT6: JP14.1 U$24.3
VCC_LGT7: JP15.1 U$25.3
VCC_LGT8: JP19.1 U$32.3
VDD1: C2.1 U$2.1(EN) U$2.2(IN) U$11.VDD
VDD2: C6.1 U$4.1(EN) U$4.2(IN) U$14.VDD

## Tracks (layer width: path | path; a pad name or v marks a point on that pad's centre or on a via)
19
  Top 0.406: R29.1 R28.1 11.41,18.4 LEFT_SWITCH.P$2
20
  Top 0.406: R31.1 R30.1 113.05,18.4 RIGHT_SWITCH.P$2
21  (via drill 0.5)
  Top 0.406: JP4.2 7.62,3.17 8.89,1.91 20.95,1.91 v22.23,3.17 | R32.1 R33.1 21.58,7 v22.23,6.98
  Bottom 0.406: v22.23,6.98 v22.23,3.17
22
  Top 0.406: JP5.2 114.95,5.7 R35.1 109.2,5.72 106.68,5.72 R34.1
!RESET
  Top 0.61: TP29.TESTPOINT J7.4 J7.3 6.35,79.25 7.62,77.98 8.89,77.98 11.57,75.3 U1.30
AIN3
  Top 0.61: LED_SWITCH.2 43.43,95.25 41.91,93.73 41.91,90.55 40.26,88.9 21.59,88.9 TP24.TESTPOINT J7.14 J7.13 19.05,78.74 16.57,76.26 U1.25
AIN4
  Top 0.61: LED_SWITCH.1 43.18,97.79 40.64,95.25 40.64,91.44 39.37,90.17 20.32,90.17 TP25.TESTPOINT J7.12 J7.11 16.51,78.74 15.57,77.8 U1.26
AIN5
  Top 0.406: TP26.TESTPOINT 14.86,87.25 14.86,93.85 16.26,95.25 HEJ3.2
  Top 0.61: U1.27 14.57,78.14 13.97,78.74 J7.9 J7.10 TP26.TESTPOINT
AIN6
  Top 0.406: HEJ2.2 12.57,95.25 13.97,93.85 13.97,88.9 TP27.TESTPOINT
  Top 0.61: U1.28 13.57,76.6 11.43,78.74 J7.7 J7.8 TP27.TESTPOINT
AIN7
  Top 0.406: TP28.TESTPOINT 7.62,87.63 7.62,93.98 6.35,95.25 HEJ1.2
  Top 0.61: U1.29 12.57,75.57 8.89,79.25 J7.5 J7.6 TP28.TESTPOINT
BATTERY
  Top 0.61: U1.31 10.57,75.03 8.89,76.71 6.35,76.71 3.81,78.74 J7.1 J7.2 TP30.TESTPOINT
BOOTLOADER_CTRL
  Top 0.61: U1.24 17.57,74.72 21.59,78.74 J7.15 J7.16 TP23.TESTPOINT
BOOTLOADER_RX
  Top 0.61: U1.22 20.47,71.27 25.4,76.2 25.4,78.74 26.67,80.01 J5.3 J5.4 TP21.TESTPOINT
BOOTLOADER_TX
  Top 0.61: U1.23 20.2,72.27 24.13,76.2 24.13,80.01 26.67,82.55 J5.1 J5.2 TP22.TESTPOINT
DEC_GEAR_SWITCH_OUT  (via drill 0.5)
  Top 0.406: R35.2 109.22,8.26 109.85,8.89 v110.49,8.89 | v111.12,4.45 110.49,3.81 C12.1 108.6,3.19 107.95,2.54 101.35,2.54 100.84,2.03 84.58,2.03 83.82,2.79 SWITCH_LEDBRKOUT.1
  Bottom 0.406: v110.49,8.89 111.12,8.26 v111.12,4.45
DGND_USB
  Top 0.61: U1.10 20.2,57.27 24.13,53.34 24.13,49.53 26.67,46.99 J3.13 J3.14 TP9.TESTPOINT
DVDD_USB
  Top 0.61: U1.13 21.01,60.27 26.67,54.61 J3.7 J3.8 TP12.TESTPOINT
GND  (via drill 0.5)
  Top 0.305: J13.5 8.89,33.76 9.4,34.27 12.73,34.27
  other vias: 12.7,38.86 14.73,31.5 28.19,31.5 48.01,30.73 58.17,67.06 72.64,67.06 26.67,86.11 34.8,86.11 22.35,97.79 25.15,64.77 22.1,31.5
  pour Bottom: 0,101.6 74.93,101.6 74.93,26.67 0,26.67
  pour Top: 0,101.6 74.93,101.6 74.93,26.67 0,26.67
GND_LEDBRKOUT  (via drill 0.5)
  other vias: 33.02,16.51 33.27,11.43 93.98,16.51 93.98,11.43
  pour Bottom: 0,24.13 127,24.13 127,0 0,0
  pour Top: 0,24.13 127,24.13 127,0 0,0
GND_LGT1  (via drill 0.3)
  other vias: 87.25,67.18
  pour Top: 76.71,69.34 94.49,69.34 94.49,64.14 76.71,64.14
  pour Bottom: 76.71,69.34 94.49,69.34 94.49,64.14 76.71,64.14
GND_LGT2  (via drill 0.3)
  other vias: 87.38,73.41
  pour Bottom: 76.71,75.56 94.49,75.56 94.49,70.36 76.71,70.36
  pour Top: 76.71,75.56 94.49,75.56 94.49,70.36 76.71,70.36
GND_LGT3  (via drill 0.3)
  other vias: 87.25,79.88
  pour Bottom: 76.71,81.91 94.49,81.91 94.49,76.96 76.71,76.96
  pour Top: 76.71,81.91 94.49,81.91 94.49,76.96 76.71,76.96
GND_LGT4  (via drill 0.3)
  other vias: 98.81,71.25
  pour Bottom: 95.63,82.17 100.97,82.17 100.97,64.26 95.63,64.26
  pour Top: 95.63,82.17 100.97,82.17 100.97,64.26 95.63,64.26
GND_LGT5  (via drill 0.3)
  other vias: 87.38,60.83
  pour Top: 76.71,62.99 94.49,62.99 94.49,57.78 76.71,57.78
  pour Bottom: 76.71,62.99 94.49,62.99 94.49,57.78 76.71,57.78
GND_LGT6  (via drill 0.3)
  other vias: 98.81,52.2
  pour Bottom: 95.63,62.87 100.97,62.87 100.97,44.96 95.63,44.96
  pour Top: 95.63,62.87 100.97,62.87 100.97,44.96 95.63,44.96
GND_LGT7  (via drill 0.3)
  other vias: 87.38,48.13
  pour Top: 76.71,50.29 94.49,50.29 94.49,45.09 76.71,45.09
  pour Bottom: 76.71,50.29 94.49,50.29 94.49,45.09 76.71,45.09
GND_LGT8  (via drill 0.3)
  other vias: 87.38,54.48
  pour Top: 76.71,56.64 94.49,56.64 94.49,51.44 76.71,51.44
  pour Bottom: 76.71,56.64 94.49,56.64 94.49,51.44 76.71,51.44
HE1GND
  Top 0.305: JP10.3 111.7,80.33 U$19.2 108.97,81.02 108.71,81.15 104.65,81.15 104.39,81.03 104.39,80.53 U$18.5
HE1OUT  (via drill 0.5)
  Top 0.305: JP10.2 110.49,77.72 109.73,76.96 109.73,75.44 109.22,74.93 105.92,74.93 105.16,75.69 R20.1 105.16,75.73 v105.16,76.96 | U$19.3 106.67,78.48 v106.43,78.23
  Bottom 0.305: v106.43,78.23 v105.16,76.96
HE1VIN
  Top 0.305: U$18.1 103.32,75.79 R20.2 103.42,74.89 103.89,74.42 109.47,74.42 110.24,75.18 JP10.1
HE2GND
  Top 0.305: U$5.5 116.97,80.9 117.22,81.15 121.54,81.15 121.79,80.9 U$12.2 124.39,80.2 JP11.3
HE2OUT  (via drill 0.5)
  Top 0.305: JP11.2 123.06,77.72 122.68,77.34 122.68,75.69 121.79,74.93 118.87,74.93 118.11,75.56 R23.1 117.82,76.67 v117.86,76.71 | v119.38,78.23 119.38,79.13 U$12.3
  Bottom 0.305: v117.86,76.71 v119.38,78.23
HE2VIN
  Top 0.305: U$5.1 116.02,75.66 R23.2 116.12,74.51 116.33,74.42 122.17,74.42 122.94,75.06 124.33,75.06 JP11.1
HE3GND
  Top 0.305: JP12.3 121.87,70.74 U$13.2 121.8,71.37 121.54,71.63 117.22,71.63 116.97,71.37 U$6.5
HE3OUT  (via drill 0.5)
  Top 0.305: JP12.2 123.06,68.2 122.68,67.82 122.68,66.17 121.92,65.41 118.87,65.41 117.98,66.29 R24.1 117.82,67.4 v117.86,67.44 | v119.38,68.58 119.38,69.6 U$13.3
  Bottom 0.305: v117.86,67.44 118.24,67.44 v119.38,68.58
HE3VIN
  Top 0.305: U$6.1 116.02,66.39 R24.2 116.12,65.11 116.33,64.9 122.3,64.9 123.06,65.66 JP12.1
HE4GND
  Top 0.305: JP9.3 109.16,70.74 U$22.2 109.1,71.24 108.71,71.63 104.52,71.63 104.27,71.37 U$21.5
HE4OUT  (via drill 0.5)
  Top 0.305: JP9.2 111.63,68.07 110.36,68.07 109.85,67.56 109.85,66.04 109.22,65.41 106.17,65.41 105.28,66.29 R38.1 105.12,67.4 v105.16,67.44 | v106.68,68.83 106.68,69.73 U$22.3
  Bottom 0.305: v105.16,67.44 105.28,67.44 v106.68,68.83
HE4VIN
  Top 0.305: U$21.1 103.32,66.39 R38.2 103.42,65.37 103.89,64.9 109.6,64.9 110.24,65.53 111.63,65.53 JP9.1
HE5GND
  Top 0.305: JP16.3 124.39,61.15 U$31.2 121.8,61.33 121.03,62.1 117.35,62.1 116.97,61.72 U$30.5
HE5OUT  (via drill 0.5)
  Top 0.305: JP16.2 123.19,58.67 122.68,58.17 122.68,56.77 121.79,55.88 118.62,55.88 117.82,56.68 R40.1 117.82,57.87 v117.86,57.91 | U$31.3 v119.5,59.19 v119.51,59.18
  Bottom 0.305: v119.51,59.18 118.24,57.91 v117.86,57.91
HE5VIN
  Top 0.305: U$30.1 116.02,56.87 R40.2 116.12,56.09 116.84,55.37 122.17,55.37 122.94,56.13 JP16.1
HE6GND
  Top 0.305: U$26.5 104.27,61.72 104.65,62.1 108.59,62.1 109.1,61.59 U$28.2 111.69,61.15 JP17.3
HE6OUT  (via drill 0.5)
  Top 0.305: R43.1 105.28,56.77 | 105.28,56.77 106.17,55.88 109.22,55.88 109.98,56.64 109.98,58.17 110.49,58.67 JP17.2 | 105.28,56.77 v105.28,57.91 | v106.68,59.18 106.68,60.08 U$28.3
  Bottom 0.305: v105.28,57.91 105.41,57.91 v106.68,59.18
HE6VIN
  Top 0.305: U$26.1 103.32,56.87 R43.2 103.42,55.84 103.89,55.37 109.47,55.37 110.24,56.13 JP17.1
HE7GND
  Top 0.305: JP18.3 124.39,51.62 U$29.2 121.8,51.94 121.16,52.58 117.35,52.58 116.97,52.2 U$27.5
HE7OUT  (via drill 0.5)
  Top 0.305: JP18.2 123.06,49.15 122.68,48.77 122.68,47.12 121.92,46.36 118.75,46.36 117.86,47.24 R44.1 117.82,48.22 v117.81,48.41 | v119.38,49.53 119.38,50.55 U$29.3
  Bottom 0.305: v117.81,48.41 118.26,48.41 v119.38,49.53
HE7VIN
  Top 0.305: U$27.1 116.02,47.34 R44.2 116.12,46.57 116.84,45.85 122.3,45.85 123.06,46.61 JP18.1
HE8GND
  Top 0.305: JP20.3 111.69,51.62 U$34.2 109.1,51.94 108.46,52.58 104.78,52.58 104.39,52.2 104.39,51.82 U$33.5
HE8OUT  (via drill 0.5)
  Top 0.305: JP20.2 110.36,49.15 109.98,48.77 109.98,47.12 109.22,46.36 106.05,46.36 105.16,47.24 R50.1 105.12,48.35 v105.16,48.39 | U$34.3 v106.8,49.66 v106.81,49.66
  Bottom 0.305: v106.81,49.66 105.54,48.39 v105.16,48.39
HE8VIN
  Top 0.305: U$33.1 103.32,47.34 R50.2 103.42,46.57 104.14,45.85 109.6,45.85 110.36,46.61 JP20.1
I2C_SCL  (via drill 1.2)
  Top 0.305: v47.88,72.39 U3.26
  Top 0.406: v47.88,72.39 47.88,80.9 53.34,86.36 53.34,93.47 53.85,93.98 LED_I2C.1
  Top 0.61: U1.17 21.82,66.27 22.86,67.31 J5.13 J5.14 TP16.TESTPOINT 39.37,63.5 R27.1
  Bottom 0.406: TP16.TESTPOINT 38.1,67.31 43.18,72.39 v47.88,72.39
I2C_SCL_LEDBRKOUT  (via drill 0.5)
  Top 0.305: v58.55,4.45 59.05,3.96 59.61,3.4 60.56,3.4 U2.26
  Bottom 0.305: I2C_LEDBRKOUT.1 73.03,4.45 v58.55,4.45
I2C_SDA
  Top 0.305: U3.27 47.24,68.98 47.24,69.98 46.1,71.12 40.64,71.12 39.37,69.85 TP17.TESTPOINT
  Top 0.406: TP17.TESTPOINT 52.07,86.36 52.07,95.25 53.34,96.52 LED_I2C.2
  Top 0.61: U1.18 21.55,67.27 24.13,69.85 J5.11 J5.12 TP17.TESTPOINT 42.16,63.25 R26.1
I2C_SDA_LEDBRKOUT  (via drill 0.5)
  Top 0.305: v58.17,3.3 58.69,2.77 U2.27
  Bottom 0.305: I2C_LEDBRKOUT.2 74.42,2.03 59.18,2.03 58.17,3.05 v58.17,3.3
INC_GEAR_SWITCH_OUT  (via drill 0.5)
  Top 0.406: C11.1 20.32,4.43 R33.2 24.15,5.7 v24.77,5.08
  Bottom 0.406: v24.77,5.08 29.21,1.27 85.09,1.27 86.36,2.54 SWITCH_LEDBRKOUT.2
LEFT_SWITCH_OUT  (via drill 0.5)
  Top 0.406: R29.2 21.59,18.43 21.59,17.15 20.95,16.51 C9.1 19.7,15.23 v20.32,14.6 | v87.63,13.34 91.44,9.52 SWITCH_LEDBRKOUT.4
  Bottom 0.406: v20.32,14.6 86.36,14.6 v87.63,13.34
N$1
  Top 0.406: RLED8.A R16.1
N$2
  Top 0.61: R6.1 R5.2 63.74,59.07 64.77,58.04 64.77,55.88 65.62,55.03 U$2.5(ADJ)
N$3
  Top 0.61: R4.1 R3.2 62.88,44.45 63.5,44.45 64.77,43.18 64.77,40.64 65.62,39.79 U$4.5(ADJ)
N$4
  Top 0.406: RLED7.A R15.1
N$5
  Top 0.406: RLED6.A R14.1
N$6
  Top 0.406: RLED5.A R13.1
N$7
  Top 0.406: RLED4.A R12.1
N$8
  Top 0.406: RLED3.A R11.1
N$9
  Top 0.406: RLED2.A R10.1
N$10
  Top 0.406: RLED1.A R9.1
N$11
  Top 0.406: GLED2.A R8.1
N$12
  Top 0.406: GLED1.A R7.1
N$13
  Top 0.305: U$22.1 109.1,67.95 108.84,67.69 108.84,66.84 R37.1
N$14
  Top 0.305: U$21.3 105.33,68.57 R37.2
N$15
  Top 0.305: R19.1 108.67,76.92 108.97,77.22 108.97,78.42 U$19.1
N$16
  Top 0.305: U$18.3 105.29,78.1 106.68,76.71 106.68,76.49 R19.2
N$17
  Top 0.305: U$31.1 121.8,58.43 121.54,58.17 121.54,57.32 R39.1
N$18
  Top 0.305: U$13.1 121.8,68.08 121.41,67.69 121.41,66.89 R21.1
N$19
  Top 0.305: U$30.3 119.69,57.28 R39.2
N$20
  Top 0.305: U$29.1 121.8,48.9 121.54,48.64 121.54,47.79 R41.1
N$21
  Top 0.305: U$6.3 118.03,68.57 R21.2
N$22
  Top 0.305: U$27.3 118.03,49.52 R41.2
N$23
  Top 0.305: R42.1 108.8,58.25 109.09,58.55 U$28.1
N$24
  Top 0.305: U$12.1 121.8,76.63 R22.1
N$25
  Top 0.305: U$5.3 117.92,77.96 R22.2
N$26
  Top 0.305: U$26.3 105.33,59.05 R42.2
N$27
  Top 0.305: U$34.1 109.1,48.9 108.84,48.64 108.84,47.79 R49.1
N$28
  Top 0.305: U$33.3 105.33,49.52 R49.2
N$29
  Top 0.305: R51.1 80.63,53.36 JP19.3
N$30
  Top 0.305: R52.1 80.63,47 JP15.3
N$31
  Top 0.305: R53.1 97.81,59.07 JP14.3
N$32
  Top 0.305: R54.1 80.63,59.7 JP13.3
N$33
  Top 0.305: R55.1 97.81,77.99 JP8.3
N$34
  Top 0.305: R56.1 80.63,78.75 JP3.3
N$35
  Top 0.406: JP6.2 109.22,88.27 INC_GEAR_SWITCH.P$4
N$36
  Top 0.406: JP6.1 INC_GEAR_SWITCH.P$2
N$37
  Top 0.305: JP7.2 93.47,88.27 DEC_GEAR_SWITCH.P$4
N$38
  Top 0.305: DEC_GEAR_SWITCH.P$2 JP7.1
N$39
  Top 0.305: R57.1 80.63,72.41 JP2.3
N$40
  pour Bottom: 77.47,100.33 100.33,100.33 100.33,83.82 77.47,83.82
N$41
  pour Top: 77.47,100.33 100.33,100.33 100.33,83.82 77.47,83.82
N$42
  Top 0.305: R58.1 80.63,66.06 JP1.3
N$43
  Top 0.305: JP21.2 109.22,31.12 INC_GEAR_SWITCH1.P$4
N$44
  Top 0.305: JP21.1 INC_GEAR_SWITCH1.P$2
N$45
  Top 0.305: JP22.2 93.98,31.12 DEC_GEAR_SWITCH1.P$4
N$46
  pour Top: 77.47,43.18 100.33,43.18 100.33,26.67 77.47,26.67
N$47
  pour Bottom: 77.47,43.18 100.33,43.18 100.33,26.67 77.47,26.67
N$48
  pour Bottom: 102.87,43.18 125.73,43.18 125.73,26.67 102.87,26.67
N$49
  Top 0.305: JP22.1 DEC_GEAR_SWITCH1.P$2
N$52  (via drill 3.2 pad 0.61)
  other vias: 38.86,19.56
N$53
  pour Bottom: 102.62,100.58 125.98,100.58 125.98,83.57 102.62,83.57
N$54
  pour Top: 102.62,100.58 125.98,100.58 125.98,83.57 102.62,83.57
N$55
  pour Top: 102.87,43.18 125.73,43.18 125.73,26.67 102.87,26.67
N$57  (via drill 3.2 pad 0.61)
  other vias: 84.58,9.91
N$58  (via drill 3.2 pad 0.61)
  other vias: 88.15,19.56
N$59  (via drill 3.2 pad 0.61)
  other vias: 42.42,9.91
N$62  (via drill 3.2 pad 0.61)
  other vias: 97.79,40.64
N$63  (via drill 3.2 pad 0.61)
  other vias: 97.79,29.21
N$64  (via drill 3.2 pad 0.61)
  other vias: 80.01,29.21
N$65  (via drill 3.2 pad 0.61)
  other vias: 80.01,40.64
N$66  (via drill 3.2 pad 0.61)
  other vias: 105.41,40.64
N$67  (via drill 3.2 pad 0.61)
  other vias: 105.41,29.21
N$69  (via drill 3.2 pad 0.61)
  other vias: 123.19,29.21
N$70  (via drill 3.2 pad 0.61)
  other vias: 123.19,40.64
N$71  (via drill 3.2 pad 0.61)
  other vias: 80.01,86.36
N$72  (via drill 3.2 pad 0.61)
  other vias: 80.01,97.79
N$73  (via drill 3.2 pad 0.61)
  other vias: 97.79,97.79
N$74  (via drill 3.2 pad 0.61)
  other vias: 97.79,86.36
N$75  (via drill 3.2 pad 0.61)
  other vias: 105.41,86.36
N$76  (via drill 3.2 pad 0.61)
  other vias: 105.41,97.79
N$77  (via drill 3.2 pad 0.61)
  other vias: 123.19,97.79
N$78  (via drill 3.2 pad 0.61)
  other vias: 123.19,86.36
N$79
  Top 0.406: R59.1 GLED4.A
OE
  Top 0.406: U3.23 49.83,70.14 50.8,71.12 52.07,71.12 53.34,72.39 53.34,73.62 R1.1
OE_LEDBRKOUT
  Top 0.305: U2.23 59.65,5.38 57.66,7.37 57.66,9.91 56.9,10.67 55.61,10.67 R2.1
OUT_LGT1
  Top 0.305: 89.57,66.13 R17.2 89.85,65.79 90.17,65.79 90.42,65.53 90.99,65.53 U$15.2 91.12,65.53 91.69,65.53 92.2,66.04 92.2,68.07 91.69,68.45 83.19,68.45 82.8,68.07 R58.2
OUT_LGT2
  Top 0.305: R25.2 U$16.2 91.11,71.88 91.69,71.88 92.2,72.39 92.2,74.3 91.57,74.68 83.06,74.68 82.8,74.42 R57.2
OUT_LGT3
  Top 0.305: R18.2 U$17.2 91.11,78.23 91.69,78.23 92.2,78.74 92.2,80.52 91.44,81.15 83.19,81.15 82.8,80.77 R56.2
OUT_LGT4
  Top 0.305: R36.2 97.41,68.78 U$20.2 97.28,67.76 97.28,67.18 97.79,66.67 99.31,66.67 100.2,67.69 100.2,75.56 99.82,75.95 R55.2 99.82,76.45
OUT_LGT5
  Top 0.305: R45.2 90.19,59.25 U$23.2 91.12,59.18 91.69,59.18 92.2,59.69 92.2,61.59 91.69,62.1 83.19,62.1 82.8,61.72 R54.2
OUT_LGT6
  Top 0.305: R47.2 97.35,49.63 U$24.2 97.28,48.71 97.28,48.01 97.66,47.62 99.57,47.62 100.2,48.26 100.2,56.52 99.82,56.9 R53.2
OUT_LGT7
  Top 0.305: R46.2 90.19,46.55 U$25.2 91.12,46.48 91.69,46.48 92.2,46.99 92.2,49.02 91.82,49.4 83.19,49.4 82.8,49.02 R52.2
OUT_LGT8
  Top 0.305: R48.2 90.19,52.9 U$32.2 91.12,52.83 91.69,52.83 92.2,53.34 92.2,55.37 91.82,55.75 83.19,55.75 82.8,55.37 R51.2
P08
  Top 0.61: TP18.TESTPOINT J5.10 J5.9 25.4,72.39 21.28,68.27 U1.19
P09
  Top 0.61: LED_SWITCH.4 45.72,85.09 TP19.TESTPOINT J5.8 J5.7 26.67,74.93 21.01,69.27 U1.20
P10
  Top 0.61: U1.21 20.74,70.27 27.94,77.47 J5.5 J5.6 TP20.TESTPOINT 43.18,85.09 43.18,91.44 44.45,92.71 LED_SWITCH.3
P17
  Top 0.61: TP1.TESTPOINT J1.1 J1.2 3.81,50.55 6.35,53.09 8.89,53.09 10.57,54.77 U1.2
P21
  Top 0.305: U4.P$11 16.51,35.56 13.97,38.1 TP5.TESTPOINT
  Top 0.61: U1.6 14.57,51.4 13.97,50.8 J1.10 J1.9 TP5.TESTPOINT
P22
  Top 0.305: U4.P$8 18.55,37.33 16.51,39.37 TP6.TESTPOINT
  Top 0.61: U1.7 15.57,51.74 16.51,50.8 J1.12 | J1.12 J1.11 | J1.12 TP6.TESTPOINT
P23
  Top 0.61: TP7.TESTPOINT J1.13 J1.14 19.05,50.8 16.57,53.28 U1.8
P24
  Top 0.61: TP8.TESTPOINT J1.15 J1.16 21.59,50.8 17.57,54.82 U1.9
PWM0
  Top 0.305: SERVO_1.3 38.1,36.83 49.78,48.51 49.78,63.08 U3.6
PWM0_0  (via drill 0.5)
  Top 0.254: R7.2 100.34,6.98 v92.71,6.98 | v90.17,6.98 88.56,5.38 U2.6
  Bottom 0.254: v92.71,6.98 v90.17,6.98
PWM1
  Top 0.305: SERVO_0.3 43.18,40.51 50.55,47.88 50.55,63.05 U3.7
PWM1_0  (via drill 0.3, 0.5)
  Top 0.254: R8.2 27.92,5.72 v34.29,5.72 | v70.76,6.02 U2.7
  Bottom 0.254: v34.29,5.72 34.59,6.02 v70.76,6.02
PWM2
  Top 0.305: BACK_LIGHTS.1 52.07,38.48 51.18,39.37 51.18,63.07 U3.8
PWM2_0  (via drill 0.3, 0.5)
  Top 0.254: R9.2 v45.72,13.34 | v68.12,6.68 v68.12,6.67 U2.8
  Bottom 0.254: v68.12,6.68 51.74,6.68 v45.72,13.34
PWM3
  Top 0.305: U3.9 51.82,63.08 51.82,40.13 54.61,37.34 54.61,35.56 53.34,34.29 BACK_LIGHTS.2
PWM3_0  (via drill 0.3, 0.5)
  Top 0.254: R10.2 v50.8,13.34 | v69.8,7.31 69.79,7.33 U2.9
  Bottom 0.254: v69.8,7.31 56.19,7.31 v50.8,13.34
PWM4
  Top 0.305: BACK_LIGHTS.3 54.61,31.75 55.88,33.02 55.88,37.47 52.45,40.89 52.45,63.1 U3.10
PWM4_0  (via drill 0.3, 0.5)
  Top 0.254: R11.2 v55.88,13.34 | v72.21,7.98 U2.10
  Bottom 0.254: v55.88,13.34 60.6,7.98 v72.21,7.98
PWM5_0  (via drill 0.3, 0.5)
  Top 0.254: R12.2 v60.96,13.34 | v74.22,8.64 74.21,8.62 U2.11
  Bottom 0.254: v60.96,13.34 65.02,8.64 v74.22,8.64
PWM6_0  (via drill 0.3, 0.5)
  Top 0.254: R13.2 67.3,13.34 v67.94,13.34 | v71.96,9.32 71.91,9.27 U2.12
  Bottom 0.254: v67.94,13.34 v71.96,9.32
PWM7_0  (via drill 0.5)
  Top 0.254: U2.13 71.14,9.92 v71.75,10.54 | v73.03,13.34 71.77,14.59 R14.2
  Bottom 0.254: v71.75,10.54 71.75,12.06 v73.03,13.34
PWM8_0  (via drill 0.5)
  Top 0.254: R15.2 77.45,13.34 v77.47,13.34 | v77.47,11.43 60.96,11.43 60.58,11.05 U2.15
  Bottom 0.254: v77.47,13.34 v77.47,11.43
PWM9_0
  Top 0.254: R16.2 79.01,12.32 59.94,12.32 58.42,10.8 58.42,10.16 58.66,9.92 U2.16
RIGHT_SWITCH_OUT  (via drill 0.5)
  Top 0.406: R31.2 105.41,18.43 105.41,17.15 106.05,16.51 C10.1 107.3,15.23 v106.68,14.6
  Bottom 0.406: v106.68,14.6 92.08,14.6 88.9,11.43 SWITCH_LEDBRKOUT.3
SIG_LGT1
  Top 0.305: JP1.2 83.19,67.44 83.82,67.94 89.92,67.94 90.42,67.56 90.99,67.56 U$15.1
SIG_LGT2
  Top 0.305: JP2.2 83.19,73.79 83.82,74.17 89.41,74.17 90.17,73.66 90.99,73.66 U$16.1
SIG_LGT3
  Top 0.305: JP3.2 83.19,80.14 83.82,80.64 90.35,80.64 U$17.1
SIG_LGT4
  Top 0.305: JP8.2 99.31,75.44 99.69,74.93 99.69,69.09 99.19,68.45 99.19,67.89 U$20.1
SIG_LGT5
  Top 0.305: JP13.2 83.19,61.09 83.69,61.59 89.92,61.59 90.3,61.21 90.99,61.21 U$23.1
SIG_LGT6
  Top 0.305: JP14.2 99.19,56.52 99.69,56.01 99.69,50.16 99.19,49.66 99.19,48.84 U$24.1
SIG_LGT7
  Top 0.305: JP15.2 83.19,48.39 83.69,48.89 89.66,48.89 90.17,48.39 90.99,48.39 U$25.1
SIG_LGT8
  Top 0.305: JP19.2 83.19,54.74 83.69,55.24 89.79,55.24 90.17,54.86 90.99,54.86 U$32.1
SPI_MISO  (via drill 0.3)
  Top 0.305: U4.P$7 19.05,38.1 20.32,39.37 22.86,39.37 v27.94,44.45
  Top 0.61: U1.14 21.28,61.27 25.4,57.15 J3.5 J3.6 TP13.TESTPOINT
  Bottom 0.305: v27.94,44.45 36.83,44.45 40.64,48.26 40.64,54.61 38.1,57.15 TP13.TESTPOINT
SPI_MOSI  (via drill 0.3)
  Top 0.305: U4.P$6 19.55,37.33 20.32,38.1 22.86,38.1 v27.94,43.18
  Top 0.61: TP14.TESTPOINT J3.4 J3.3 24.26,59.69 21.68,62.27 U1.15
  Bottom 0.305: v27.94,43.18 36.83,43.18 41.91,48.26 41.91,55.88 38.1,59.69 TP14.TESTPOINT
SPI_SCK  (via drill 0.3)
  Top 0.305: U4.P$4 22.09,36.06 v27.94,41.91
  Top 0.61: U1.16 21.82,63.27 22.86,62.23 J3.1 J3.2 TP15.TESTPOINT
  Bottom 0.305: v27.94,41.91 36.83,41.91 43.18,48.26 43.18,57.15 38.1,62.23 TP15.TESTPOINT
TCK
  Top 0.305: J13.4 7.62,34.98 6.63,35.97 6.63,39.47 8.89,41.73 TP3.TESTPOINT
  Top 0.61: TP3.TESTPOINT J1.5 J1.6 8.89,50.29 12.57,53.97 U1.4
TDO
  Top 0.305: J13.6 8.89,35.38 11.43,37.92 TP4.TESTPOINT
  Top 0.61: TP4.TESTPOINT J1.7 J1.8 11.43,50.8 13.57,52.94 U1.5
TMS
  Top 0.305: J13.2 6.27,34.92 5.84,35.36 3.3,35.36 2.59,35.81 2.59,38.18 6.35,41.94 TP2.TESTPOINT
  Top 0.61: TP2.TESTPOINT J1.3 J1.4 6.35,50.8 7.62,51.82 9.14,51.82 11.57,54.24 U1.3
USB_N
  Top 0.61: TP11.TESTPOINT J3.10 J3.9 27.94,52.07 20.74,59.27 U1.12
USB_P
  Top 0.61: U1.11 20.47,58.27 25.4,53.34 25.4,50.8 26.67,49.53 J3.11 J3.12 TP10.TESTPOINT
VCC(3.3V)  (via drill 0.5 pad 0.61, 1.2)
  Top 0.305: 18.54,33.78 18.55,33.79 U4.P$14 | 20.93,34.52 20.44,34.52 U4.P$1
  Top 0.406: 46.1,68.96 U3.28 | J13.1 6.35,33.02 6.66,32.72 6.66,29.29 7.21,28.73 7.49,28.73 | 7.49,28.73 7.62,28.73 | 7.62,28.73 17.83,28.73 18.31,29.21 C5.1 | 7.47,28.7 7.49,28.73 | 7.62,28.73 7.59,28.7 3.81,28.7 1.4,31.12 1.4,38.99 v2.67,40.26 | C5.1 C4.1 18.54,31.82 18.54,33.78 | C5.1 18.62,28.58 18.9,28.3 22.39,28.3 23.88,29.78 23.88,33.08 22.44,34.52 20.93,34.52 | v2.29,77.22 2.29,75.04 R59.2
  Top 0.61: R6.2 58.42,55.56 C7.1 59.88,53.85 58.93,53.85 v55.88,50.8 | R27.2 R26.2 42.33,54.99 v44.96,54.99 | 46.1,68.96 45.46,68.96 44.96,68.45 v44.96,54.99 | v44.96,54.99 47.43,54.99 C3.1 | U$2.4(OUT) 67.98,56.77 71.12,56.77 72.39,58.04 72.39,62.23 64.77,69.85 59.69,69.85 55.88,73.66 55.88,80.01 v53.34,82.55 | U1.1 8.49,54.61 4.7,54.61 v2.94,52.85 1.4,51.31 1.4,41.53 v2.67,40.26
  Bottom 0.406: v2.94,52.85 2.94,53.02 2.36,53.59 2.36,77.14 v2.29,77.22
  Bottom 0.61: v55.88,50.8 48.26,50.8 | 48.26,50.8 44.96,52.83 v44.96,54.99 | v53.34,82.55 44.45,82.55 36.83,90.17 LED_VCC.1 | LED_VCC.1 34.29,90.17 20.32,90.17 HEJ3.1 HEJ2.1 HEJ1.1 | LED_VCC.1 LED_VCC.2 LED_VCC.3 | 48.26,50.8 37.72,40.26 v2.67,40.26
  Bottom 1.27: U$2.4(OUT) 61.81,56.73 v55.88,50.8
VCC(6V)  (via drill 1.2)
  Top 0.61: R4.2 58.42,40.64 60.01,39.05 C8.1 59.76,38.48 57.4,38.48 55.13,40.75 v55.13,41.49
  Bottom 1.27: U$4.4(OUT) v55.13,41.49 50.38,41.49 48.26,39.37 48.26,35.56 46.99,34.29 SERVO_0.2 SERVO_1.2
VCC_LEDBRKOUT  (via drill 0.5)
  Top 0.254: U2.28 U2.1
  Top 0.406: R28.2 17.78,20.95 19.05,22.23 20.95,22.23 22.86,20.32 v22.86,12.7 21.59,11.43 19.05,11.43 16.51,8.89 16.51,6.35 17.16,5.7 R32.2 | R30.2 109.22,21.59 108.59,22.23 105.41,22.23 104.14,20.95 v104.14,9.54 R34.2 | v101.6,1.52 51.82,1.52 VCC_LEDBRKOUT.2 | VCC_LEDBRKOUT.3 53.02,2.86 C1.1 56.62,2.12 U2.28
  Bottom 0.406: v22.86,12.7 33.66,1.91 45.09,1.91 VCC_LEDBRKOUT.1 VCC_LEDBRKOUT.2 VCC_LEDBRKOUT.3 | v104.14,9.54 104.14,3.43 v101.6,1.52
VCC_LGT1
  Top 0.305: U$15.3 92.59,64.9 86.74,64.9 JP1.1
VCC_LGT2
  Top 0.305: U$16.3 92.97,71.76 92.71,71.25 86.61,71.25 JP2.1
VCC_LGT3
  Top 0.305: U$17.3 92.59,77.6 92.46,77.6 86.61,77.6 JP3.1
VCC_LGT4
  Top 0.305: U$20.3 96.65,66.54 96.65,71.75 JP8.1
VCC_LGT5
  Top 0.305: JP13.1 85.85,59.69 87,58.55 92.46,58.55 93.34,59.44 U$23.3
VCC_LGT6
  Top 0.305: JP14.1 96.65,52.7 96.65,47.24 97.29,46.48 U$24.3
VCC_LGT7
  Top 0.305: JP15.1 86.87,45.85 92.84,45.85 93.35,46.36 U$25.3
VCC_LGT8
  Top 0.305: JP19.1 85.85,53.34 87,52.2 92.84,52.2 93.34,52.7 U$32.3
VDD1
  Top 0.61: U$2.1(EN) 62.94,61.84 C2.1
  Bottom 1.27: U$11.VDD 66.69,92.72 64.52,90.55 64.52,89.92 57.15,82.55 57.15,72.63 U$2.1(EN) U$2.2(IN)
VDD2
  Top 0.61: U$4.1(EN) 65.16,46.6 63.5,48.26 C6.1
  Bottom 1.27: U$14.VDD 66.69,77.36 64.14,74.8 64.14,70.48 72.39,62.23 72.39,51.04 U$4.1(EN) U$4.2(IN)

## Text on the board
tPlace: SDA | SCL | A | SmartBike | Ambe, Hardin, / Kenny, Singh, Zhen | 11/5/2015 | D | I | R | L | A | SCL | SDA | D.A., C.H., / T.K., K.S., / A.Z.

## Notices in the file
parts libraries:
SparkFun-Sensors: Licensing: CC v3.0 Share-Alike You are welcome to use this library for commercial purposes.
